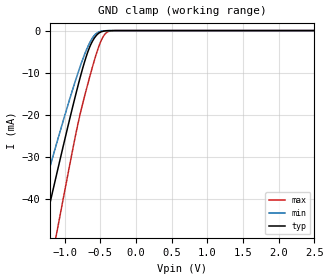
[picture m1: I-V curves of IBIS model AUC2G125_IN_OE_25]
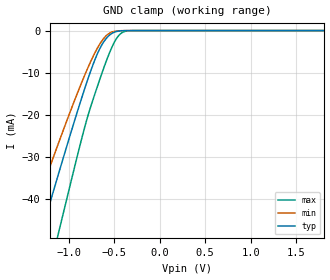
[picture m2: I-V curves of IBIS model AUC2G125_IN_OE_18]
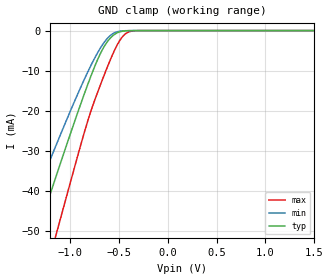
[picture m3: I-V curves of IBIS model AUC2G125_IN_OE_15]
| TEXAS INSTRUMENTS INCORPORATED
| Standard Linear and Logic Group
| IBIS Model of SN74AUC2G125
| Dual Bus Buffer Gate With 3-State Outputs
| This file contains package information for the following:
|  TSSOP 8-pin (DCT) package as [Component] AUC2G125_DCT
|  TSSOP 8-pin (DCU) package as [Component] AUC2G125_DCU
|  DSBGA 8-pin (YEP) package as [Component] AUC2G125_YEP
|  DSBGA 8-pin (YZP) package as [Component] AUC2G125_YZP
| This device can be powered at the following Vccs:
|  2.5 volt Vcc
|  1.8 volt Vcc
|  1.5 volt Vcc
|  1.2 volt Vcc
|  0.8 volt Vcc
| This file provides unique models under the [Model Selector] for each Vcc.
| For operation at a specific Vcc, select the appropriate model after each
| [Model Selector] keyword.
[IBIS Ver]   3.2
[Comment char]  |_char
[File Name]   sn74auc2g125.ibs
[File Rev]   1.2 | a_die
[Date]   January 27, 2004
[Source]   Data created from TI-SPICE simulations at TI-SLL.
[Notes]   The following is an IBIS list for the AUC2G125.
   Please contact sllibis@ti.com with questions and
   comments concerning SLL IBIS models.
   - Power clamp data deleted as there is no power-clamp diode.
   - End point warning due to AC and DC mismatch.
   - Non-monotonic data in pullup and pulldown due to
   feedback circuit.
   - FILE REV HISTORY
   - 1.2 added YEP and YZP packages on 01/27/04
[Disclaimer] Property of Texas Instruments Incorporated.  Unauthorized
   reproduction and/or distribution is strictly prohibited.
   This product is protected under copyright law.
   Created  2003, (C) Copyright  2003, Texas Instruments
   Incorporated, All Rights Reserved
   UNLESS THERE IS A SIGNED, WRITTEN AGREEMENT TO THE
   CONTRARY, TEXAS INSTRUMENTS (TI) IS PROVIDING THE IBIS
   MODELS  AND WITHOUT ANY WARRANTY, EXPRESSED OR
   IMPLIED.  TI assumes no liability for:
   1) the accuracy of the IBIS models provided to your
   company;
   2) the proper functioning of these IBIS Models in your
   design or for any resulting applications; or
   3) infringement of patents, copyrights or intellectual
   property rights resulting from your use of these IBIS
   models.
   TI provides IBIS Models as a service to our customers.
   You and your company shall not distribute, sell or give
   these models to anyone else without prior written
   permission from TI.
   TI reserves the right to make changes to our products or
   to discontinue any semiconductor product or service
   without notice, and advises our customers to obtain the
   latest version of relevant information to verify, before
   placing orders, that the information being relied on is
   current.
   Please be aware that your receipt and use of the IBIS
   information provided shall serve as acceptance of these
   terms and conditions.  If you do not accept these terms,
   you should return or destroy the IBIS models and any
   other accompanying information immediately.
| Component AUC2G125_DCT 8-pin TSSOP
[Component]   AUC2G125_DCT
[Manufacturer]   Texas Instruments, Inc.
[Package]
|   typ   min   max
R_pkg   2.900e-02   2.800e-02   3.100e-02
L_pkg   1.796e-09   1.666e-09   1.924e-09
C_pkg   1.090e-13   8.300e-14   1.360e-13
[Pin]   signal_name   model_name   R_pin   L_pin   C_pin
1   1NOE   AUC2G125_IN_OE   3.100e-02   1.894e-09   1.340e-13
2   1A   AUC2G125_IN   2.800e-02   1.697e-09   8.600e-14
3   2Y   AUC2G125_OUT   3.000e-02   1.722e-09   8.600e-14
4   GND   GND   3.000e-02   1.861e-09   1.300e-13
5   2A   AUC2G125_IN   2.800e-02   1.924e-09   1.360e-13
6   1Y   AUC2G125_OUT   2.900e-02   1.736e-09   8.600e-14
7   2NOE   AUC2G125_IN_OE   2.800e-02   1.666e-09   8.300e-14
8   VCC   POWER   3.000e-02   1.871e-09   1.320e-13
| Component AUC2G125_DCU 8-pin TSSOP
[Component]   AUC2G125_DCU
[Manufacturer]   Texas Instruments, Inc.
[Package]
|   typ   min   max
R_pkg   1.400e-02   1.300e-02   1.500e-02
L_pkg   1.289e-09   1.025e-09   2.014e-09
C_pkg   1.360e-13   6.600e-14   2.940e-13
[Pin]   signal_name   model_name   R_pin   L_pin   C_pin
1   1NOE   AUC2G125_IN_OE   1.400e-02   1.387e-09   1.760e-13
2   1A   AUC2G125_IN   1.300e-02   1.026e-09   6.600e-14
3   2Y   AUC2G125_OUT   1.300e-02   1.032e-09   6.700e-14
4   GND   GND   1.500e-02   2.014e-09   2.940e-13
5   2A   AUC2G125_IN   1.400e-02   1.412e-09   1.780e-13
6   1Y   AUC2G125_OUT   1.300e-02   1.030e-09   6.600e-14
7   2NOE   AUC2G125_IN_OE   1.300e-02   1.025e-09   6.600e-14
8   VCC   POWER   1.400e-02   1.386e-09   1.760e-13
| Component AUC2G125_YEP 8-pin DSBGA
[Component]   AUC2G125_YEP
[Manufacturer]   Texas Instruments, Inc.
[Package]
|   typ   min   max
R_pkg   1.000e-03   1.000e-03   1.000e-03
L_pkg   2.450e-11   2.400e-11   2.500e-11
C_pkg   6.550e-14   6.400e-14   6.700e-14
[Pin]   signal_name   model_name   R_pin   L_pin   C_pin
1   1NOE   AUC2G125_IN_OE   1.000e-03   2.500e-11   6.400e-14
2   1A   AUC2G125_IN   1.000e-03   2.400e-11   6.700e-14
3   2Y   AUC2G125_OUT   1.000e-03   2.400e-11   6.700e-14
4   GND   GND   1.000e-03   2.500e-11   6.400e-14
5   2A   AUC2G125_IN   1.000e-03   2.500e-11   6.400e-14
6   1Y   AUC2G125_OUT   1.000e-03   2.400e-11   6.700e-14
7   2NOE   AUC2G125_IN_OE   1.000e-03   2.400e-11   6.700e-14
8   VCCB   POWER   1.000e-03   2.500e-11   6.400e-14
| Component AUC2G125_YZP 8-pin DSBGA
[Component]   AUC2G125_YZP
[Manufacturer]   Texas Instruments, Inc.
[Package]
|   typ   min   max
R_pkg   1.000e-03   1.000e-03   1.000e-03
L_pkg   2.450e-11   2.400e-11   2.500e-11
C_pkg   6.550e-14   6.400e-14   6.700e-14
[Pin]   signal_name   model_name   R_pin   L_pin   C_pin
1   1NOE   AUC2G125_IN_OE   1.000e-03   2.500e-11   6.400e-14
2   1A   AUC2G125_IN   1.000e-03   2.400e-11   6.700e-14
3   2Y   AUC2G125_OUT   1.000e-03   2.400e-11   6.700e-14
4   GND   GND   1.000e-03   2.500e-11   6.400e-14
5   2A   AUC2G125_IN   1.000e-03   2.500e-11   6.400e-14
6   1Y   AUC2G125_OUT   1.000e-03   2.400e-11   6.700e-14
7   2NOE   AUC2G125_IN_OE   1.000e-03   2.400e-11   6.700e-14
8   VCCB   POWER   1.000e-03   2.500e-11   6.400e-14
| Model AUC2G125_IN_OE
[Model Selector]   AUC2G125_IN_OE
AUC2G125_IN_OE_25   2.5 volt Vcc
AUC2G125_IN_OE_18   1.8 volt Vcc
AUC2G125_IN_OE_15   1.5 volt Vcc
AUC2G125_IN_OE_12   1.2 volt Vcc
AUC2G125_IN_OE_08   0.8 volt Vcc
| Model AUC2G125_IN
[Model Selector]   AUC2G125_IN
AUC2G125_IN_25   2.5 volt Vcc
AUC2G125_IN_18   1.8 volt Vcc
AUC2G125_IN_15   1.5 volt Vcc
AUC2G125_IN_12   1.2 volt Vcc
AUC2G125_IN_08   0.8 volt Vcc
| Model AUC2G125_OUT
[Model Selector]   AUC2G125_OUT
AUC2G125_OUT_25   2.5 volt Vcc
AUC2G125_OUT_18   1.8 volt Vcc
AUC2G125_OUT_15   1.5 volt Vcc
AUC2G125_OUT_12   1.2 volt Vcc
AUC2G125_OUT_08   0.8 volt Vcc
| Models and submodels in the file (15): AUC2G125_IN_OE_25 (Input), AUC2G125_IN_OE_18 (Input), AUC2G125_IN_OE_15 (Input), AUC2G125_IN_OE_12 (Input), AUC2G125_IN_OE_08 (Input), AUC2G125_IN_25 (Input), AUC2G125_IN_18 (Input), AUC2G125_IN_15 (Input), AUC2G125_IN_12 (Input), AUC2G125_IN_08 (Input), AUC2G125_OUT_25 (3-state), AUC2G125_OUT_18 (3-state), AUC2G125_OUT_15 (3-state), AUC2G125_OUT_12 (3-state), AUC2G125_OUT_08 (3-state)
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[Model]   AUC2G125_IN_OE_25
Model_type  Input
Vinl=0.7
Vinh=1.7
| variable   typ   min   max
C_comp   2.55pF   1.99pF   2.92pF
[Temperature Range]   40   100   -40
| Ambient temperature   25   85   -40
[Voltage range]   2.5   2.3   2.7
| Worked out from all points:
|   GND clamp passes 1 mA (typ) near -0.55 V on its own axis
[GND Clamp]
| AUC2G125_IN_OE_25
|   Voltage   I(typ)   I(min)   I(max)
-3.6V     -223.1mA   -186.8mA   -268.3mA
-1.485V   -62.1mA    -49.68mA   -81.81mA
-1.435V   -58.34mA   -46.58mA   -77.34mA
-1.3V     -48.22mA   -38.26mA   -65.26mA
-1.115V   -34.53mA   -27.12mA   -48.68mA
-830mV    -14.34mA   -11.03mA   -23.64mA
-720mV    -7.475mA   -5.71mA    -15.68mA
-625mV    -3.066mA   -2.194mA   -9.633mA
-525mV    -682.6uA   -365uA     -4.021mA
-430mV    -73.19uA   -35.15uA   -776.9uA
-325mV    -3.339uA   -2.023uA   -30.74uA
2.5V      328.6pA    416.1pA    485.4pA
[Model]   AUC2G125_IN_OE_18
Model_type  Input
Vinl=0.5775
Vinh=1.2675
| variable   typ   min   max
C_comp   2.60pF   2.12pF   3.01pF
[Temperature Range]   40   100   -40
| Ambient temperature   25   85   -40
[Voltage range]   1.8   1.65   1.95
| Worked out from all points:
|   GND clamp passes 1 mA (typ) near -0.55 V on its own axis
[GND Clamp]
| AUC2G125_IN_OE_18
|   Voltage   I(typ)   I(min)   I(max)
-3.6V     -223.1mA   -186.8mA   -268.3mA
-1.475V   -61.35mA   -49.06mA   -80.92mA
-1.43V    -57.96mA   -46.27mA   -76.89mA
-1.295V   -47.84mA   -37.96mA   -64.81mA
-1.145V   -36.73mA   -28.9mA    -51.37mA
-1.095V   -33.06mA   -25.94mA   -46.89mA
-830mV    -14.34mA   -11.03mA   -23.64mA
-685mV    -5.613mA   -4.259mA   -13.41mA
-560mV    -1.272mA   -762.6uA   -5.827mA
-485mV    -290.6uA   -142.1uA   -2.305mA
-420mV    -55.81uA   -27.03uA   -608.5uA
1.8V      213.9pA    308.4pA    246.3pA
[Model]   AUC2G125_IN_OE_15
Model_type  Input
Vinl=0.49
Vinh=1.04
| variable   typ   min   max
C_comp   2.62pF   2.19pF   3.01pF
[Temperature Range]   40   100   -40
| Ambient temperature   25   85   -40
[Voltage range]   1.5   1.4   1.6
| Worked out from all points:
|   GND clamp passes 1 mA (typ) near -0.55 V on its own axis
[GND Clamp]
| AUC2G125_IN_OE_15
|   Voltage   I(typ)   I(min)   I(max)
-3.6V     -223.1mA   -186.8mA   -268.3mA
-1.505V   -63.61mA   -50.93mA   -83.59mA
-1.46V    -60.22mA   -48.13mA   -79.57mA
-1.325V   -50.08mA   -39.79mA   -67.5mA
-1.17V    -38.57mA   -30.39mA   -53.61mA
-1.12V    -34.89mA   -27.41mA   -49.13mA
-840mV    -15.01mA   -11.55mA   -24.46mA
-695mV    -6.121mA   -4.657mA   -14.06mA
-570mV    -1.488mA   -922uA     -6.381mA
-430mV    -73.19uA   -35.15uA   -776.9uA
-280mV    -781.4nA   -560.5nA   -5.358uA
1.5V      174.7pA    268pA      181.1pA
